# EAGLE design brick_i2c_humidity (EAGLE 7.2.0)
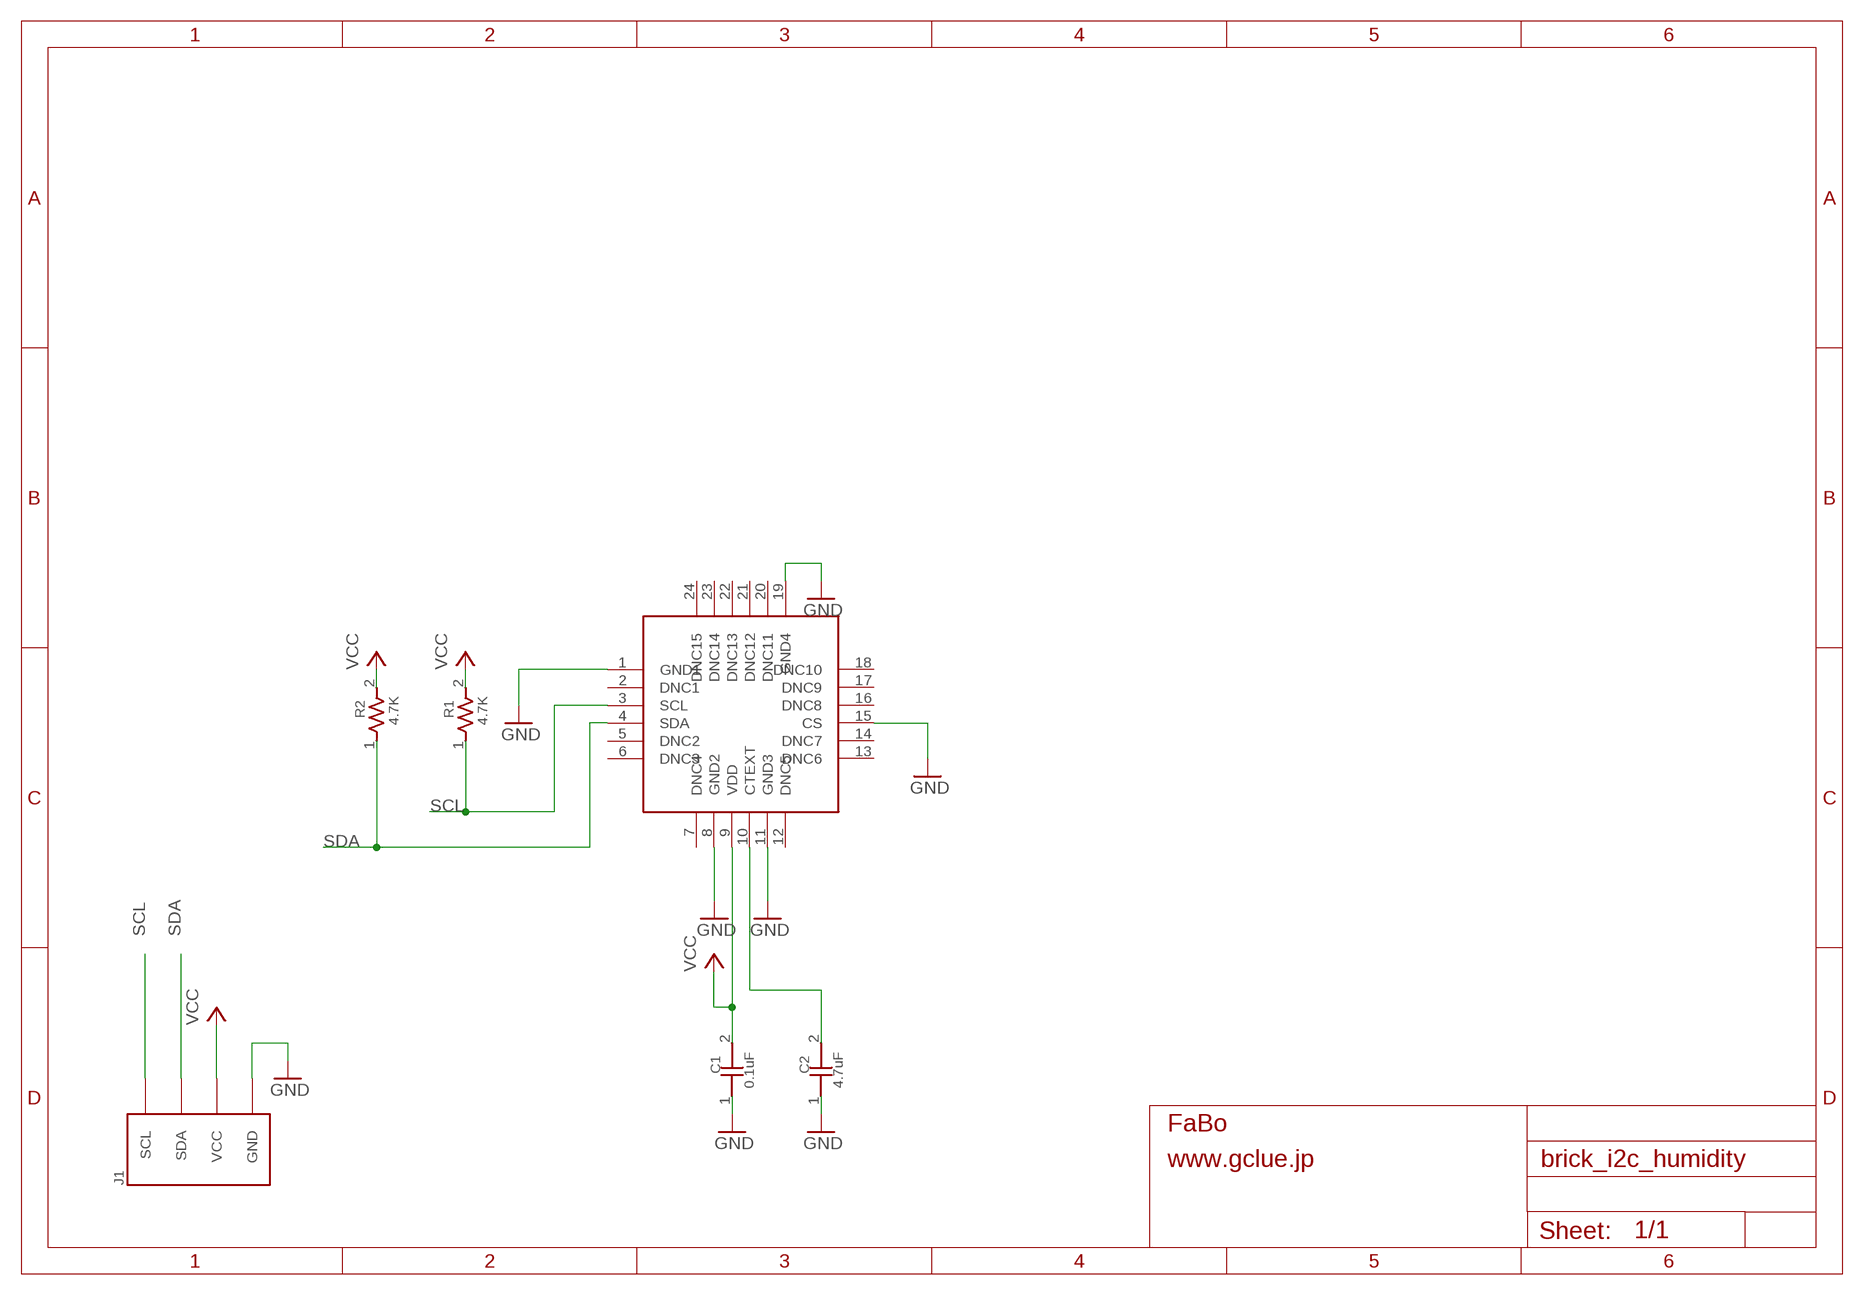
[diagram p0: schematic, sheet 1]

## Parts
C1  0.1uF  CAPACITOR0603  [0603]
C2  4.7uF  CAPACITOR0603  [0603]
J1  BRICK_I2C  [BRICK_I2C]
R1  4.7K  RESISTOR0603  [0603]
R2  4.7K  RESISTOR0603  [0603]
SI1  SILICONLAB-SI7005  [SILICONLAB-SI7005]

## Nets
GND: C1.1 C2.1 J1.GND SI1.1(GND1) SI1.8(GND2) SI1.11(GND3) SI1.15(CS) SI1.19(GND4)
N$1: C2.2 SI1.10(CTEXT)
SCL: J1.SCL R1.1 SI1.3(SCL)
SDA: J1.SDA R2.1 SI1.4(SDA)
VCC: C1.2 J1.VCC R1.2 R2.2 SI1.9(VDD)
Unconnected: SI1.2(DNC1) SI1.5(DNC2) SI1.6(DNC3) SI1.7(DNC4) SI1.12(DNC5) SI1.13(DNC6) SI1.14(DNC7) SI1.16(DNC8) SI1.17(DNC9) SI1.18(DNC10) SI1.20(DNC11) SI1.21(DNC12) SI1.22(DNC13) SI1.23(DNC14) SI1.24(DNC15)

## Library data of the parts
C1 C2 = GClue-Capacitor:CAPACITOR
J1 = gclue:BRICK_I2C: FaBo Brick 4pin(I2C)
R1 R2 = GClue-Resistors:RESISTOR
SI1 = gclueSensor:SILICONLAB-SI7005

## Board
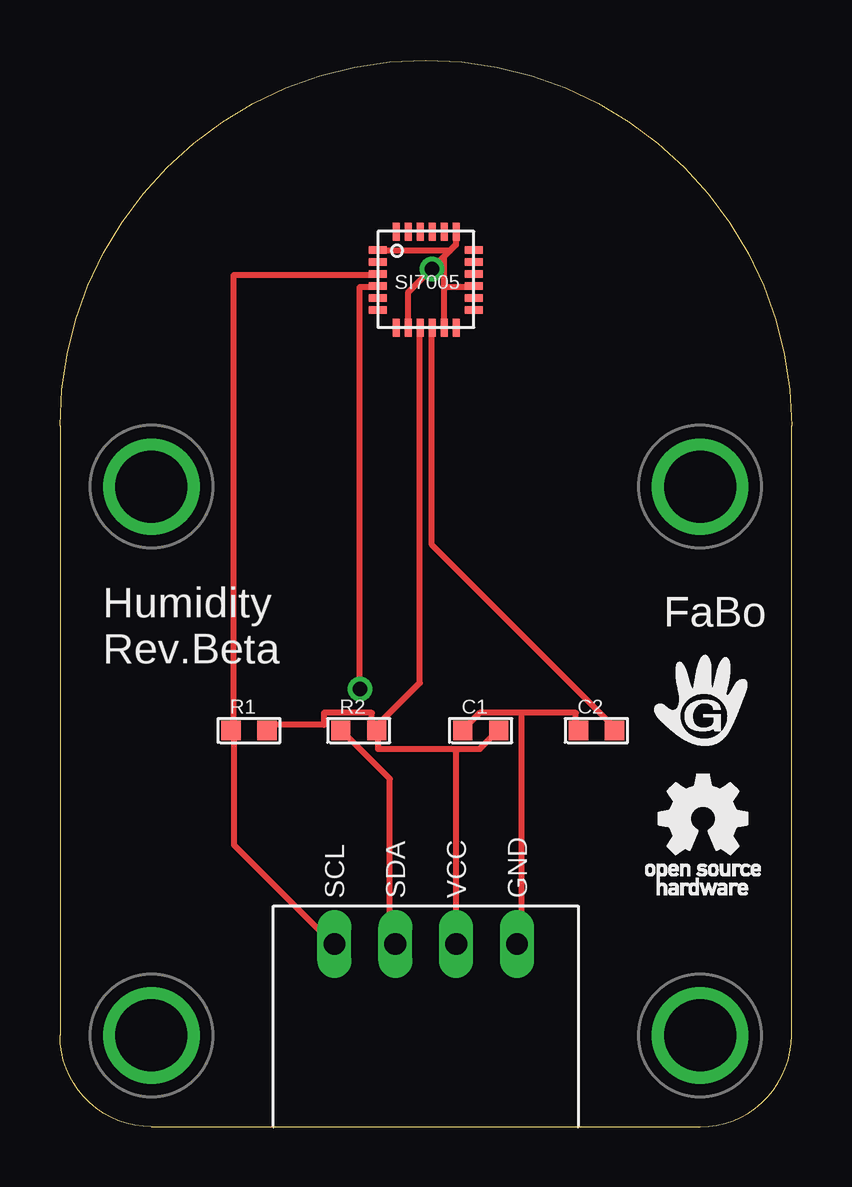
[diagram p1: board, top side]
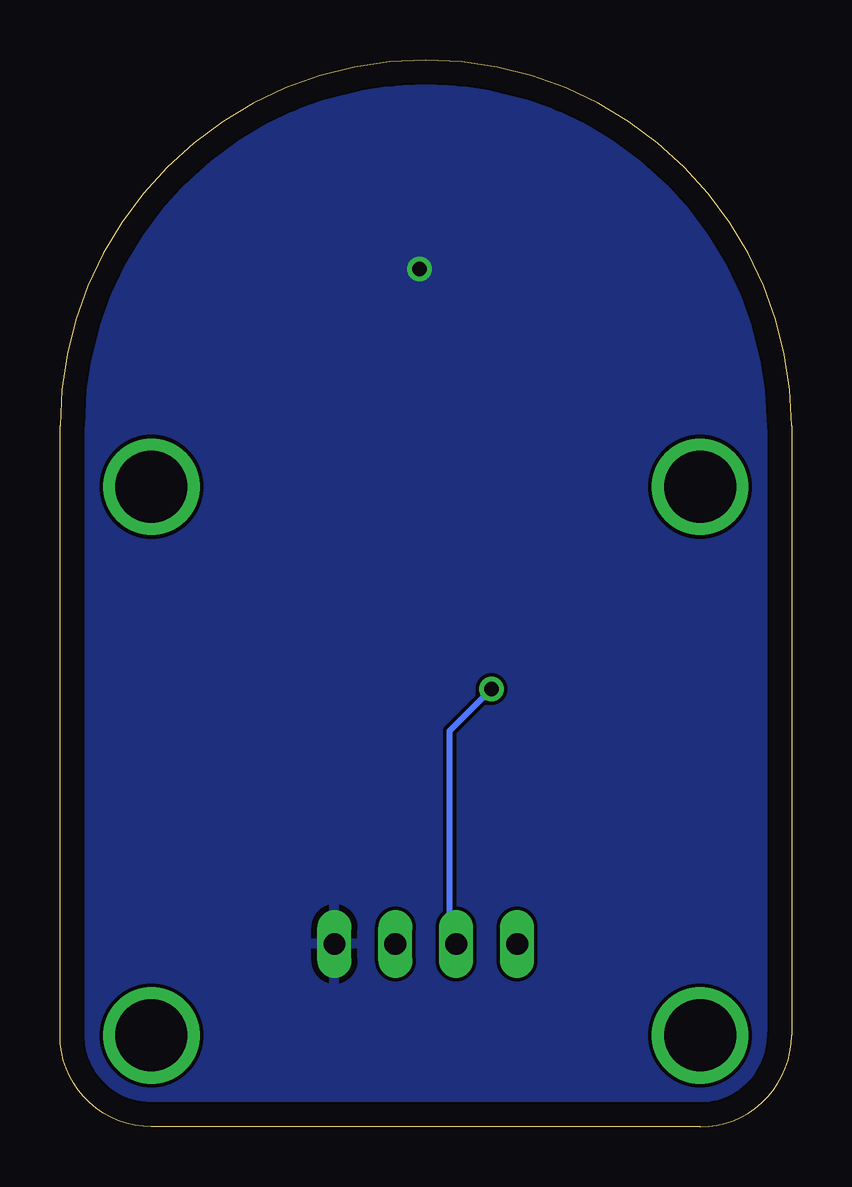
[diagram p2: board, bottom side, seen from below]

Size 30.48 x 44.45 mm. Coordinates in mm from the lower left corner, seen from the top.
Copper layers (1*16): Top 0.035mm / dielectric 1.5mm / Bottom 0.035mm
Design rules "default *": minimum track width 10mil, minimum drill 24mil, track to track 6mil, track to pad 6mil, pad to pad 6mil, via to via 6mil, smd to smd 6mil, copper to edge 40mil, drill to drill 8mil, minimum pad ring 10mil, minimum via ring 8mil, stop-mask expansion 4mil, vias tented up to drill 0mil, thermal gap 10mil

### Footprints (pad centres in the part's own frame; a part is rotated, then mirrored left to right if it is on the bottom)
0603 = smd 0.8 x 0.8: 1 -0.75,0; 2 0.75,0
BRICK_I2C = drill 0.9 long: GND 3.81,-11.43; SCL -3.81,-11.43; SDA -1.27,-11.43; VCC 1.27,-11.43 | drill 3 pad 3.81: P$5 -11.43,7.62; P$6 11.43,7.62; P$7 -11.43,-15.24; P$8 11.43,-15.24
SILICONLAB-SI7005 = smd 0.75 x 0.3: 1 -2.01,1.23; 2 -2.01,0.73; 3 -2.01,0.23; 4 -2.01,-0.27; 5 -2.01,-0.77; 6 -2.01,-1.27; 13 1.99,-1.27; 14 1.99,-0.77; 15 1.99,-0.27; 16 1.99,0.23; 17 1.99,0.73; 18 1.99,1.23 | smd 0.3 x 0.75: 7 -1.23,-2.01; 8 -0.73,-2.01; 9 -0.23,-2.01; 10 0.27,-2.01; 11 0.77,-2.01; 12 1.27,-2.01; 19 1.27,1.99; 20 0.77,1.99; 21 0.27,1.99; 22 -0.23,1.99; 23 -0.73,1.99; 24 -1.23,1.99

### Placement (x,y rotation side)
C1  17.53,16.51 0 top
C2  22.35,16.51 0 top
J1  15.24,19.05 0 top
R1  7.87,16.51 0 top
R2  12.45,16.51 0 top
SI1  15.24,35.31 0 top
U$2  [LOGO_GCLUE_M]  26.67,17.78 0 top
U$3  [LOGO_OSHW_T_M]  26.92,12.19 0 top

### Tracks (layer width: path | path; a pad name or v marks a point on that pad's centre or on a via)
GND  (via drill 0.61)
  Top 0.254: 16.25,36.5 16.5,36.75 16.5,37.25 SI1.19 | 16.25,36.5 16,36.25 | 16,36.25 v15.5,35.75 14.5,34.75 14.5,33.5 SI1.8 | 16,36.25 16,35 | 16,35 16,33.5 SI1.11 | 16,35 17,35 SI1.15 | 16.25,36.5 13.25,36.5 SI1.1 | 19.25,17.25 21.5,17.25 21.5,16.75 C2.1 | 19.25,17.25 17.5,17.25 17,16.75 C1.1 | 19.25,17.25 19.25,7.75 J1.GND
  pour Bottom: -0.25,-0.25 30.73,0 30.99,45.21 -0.51,44.7
N$1
  Top 0.254: SI1.10 15.5,33.25 15.5,24.25 23,16.75 C2.2
SCL
  Top 0.254: SI1.3 13,35.5 7.25,35.5 7.25,16.75 R1.1 7.25,16.5 7.25,11.75 11.25,7.75 J1.SCL
SDA  (via drill 0.61)
  Top 0.254: v12.5,18.25 12.5,35 13,35 SI1.4 | R2.1 11.75,16.5 13.75,14.5 13.75,7.75 J1.SDA
  Bottom 0.254: v12.5,18.25 14.25,16.5 14.25,7.75 14,7.75 J1.SDA
VCC
  Top 0.254: SI1.9 15,33.25 15,18.5 13.25,16.75 R2.2 | R1.2 8.75,16.75 11,16.75 11,17.25 13,17.25 13,16.75 R2.2 | 16.5,15.75 13.25,15.75 13.25,16.5 R2.2 | 16.5,15.75 17.5,15.75 18.25,16.5 C1.2 | 16.5,15.75 16.5,7.75 J1.VCC

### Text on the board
tPlace: FaBo | Humidity / Rev.Beta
